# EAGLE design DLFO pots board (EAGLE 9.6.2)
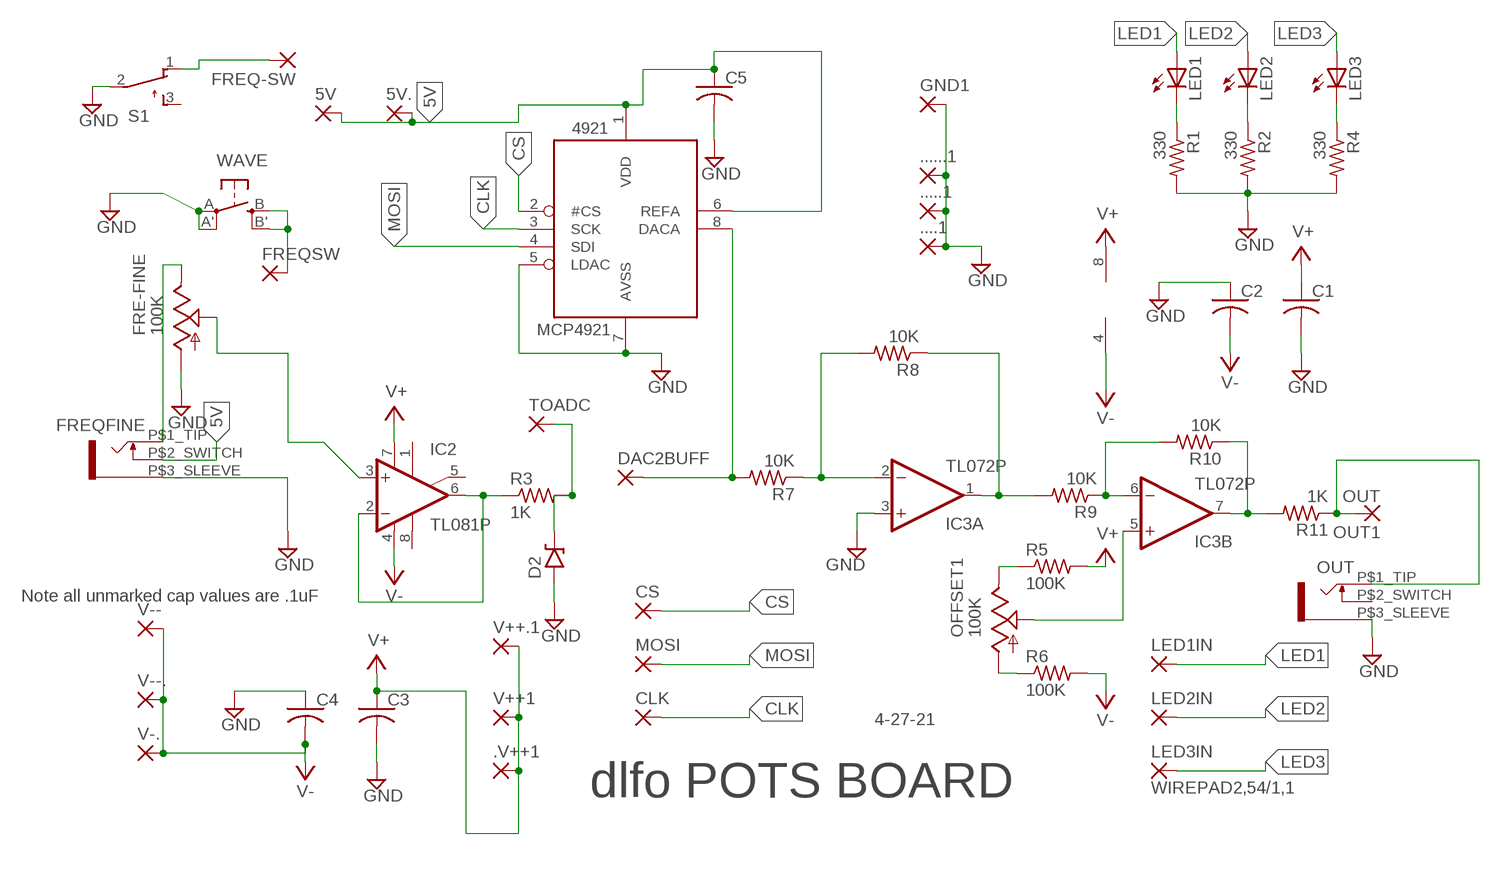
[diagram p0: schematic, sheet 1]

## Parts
5V  2,54/1,0  [2,54/1,0]
5V.  2,54/1,0  [2,54/1,0]
4921  MCP4921  [DIL08]
....1  3,17/1,3  [3,17/1,3]
.....1  3,17/1,3  [3,17/1,3]
......1  3,17/1,3  [3,17/1,3]
.V++1  2,54/1,0  [2,54/1,0]
C1  C-US025-024X044  [C025-024X044]
C2  C-US025-024X044  [C025-024X044]
C3  C-US025-024X044  [C025-024X044]
C4  C-US025-025X050  [C025-025X050]
C5  C-US025-024X044  [C025-024X044]
CLK  WIREPAD2,54/1,1  [2,54/1,1]
CS  2,54/1,0  [2,54/1,0]
D2  ZENER.2  [DO41-2]
DAC2BUFF  3,17/1,3  [3,17/1,3]
FRE-FINE  100K  9MM_SNAP-IN_POT_  [9MM_SNAP-IN_POT]
FREQ-SW  2,54/1,0  [2,54/1,0]
FREQFINE  WQP-PJ301M-12_JACK  [WQP-PJ301M-12_JACK]
FREQSW  2,54/1,0  [2,54/1,0]
GND1  3,17/1,3  [3,17/1,3]
IC2  TL081P  [DIL08@1]
IC3  TL072P  [DIL08]
LED1  LED3MM  [LED3MM]
LED1IN  2,54/1,0  [2,54/1,0]
LED2  LED3MM  [LED3MM]
LED2IN  2,54/1,0  [2,54/1,0]
LED3  LED3MM  [LED3MM]
LED3IN  WIREPAD2,54/1,1  [2,54/1,1]
MOSI  2,54/1,0  [2,54/1,0]
OFFSET1  100K  9MM_SNAP-IN_POT_  [9MM_SNAP-IN_POT]
OUT  WQP-PJ301M-12_JACK  [WQP-PJ301M-12_JACK]
OUT1  OUT  3,17/1,3  [3,17/1,3]
R1  330  R-US_0204/7  [0204/7]
R2  330  R-US_0204/7  [0204/7]
R3  1K  R-US_0204/7  [0204/7]
R4  330  R-US_0204/7  [0204/7]
R5  100K  R-US_0204/7  [0204/7]
R6  100K  R-US_0204/7  [0204/7]
R7  10K  R-US_0204/7  [0204/7]
R8  10K  R-US_0204/7  [0204/7]
R9  10K  R-US_0204/7  [0204/7]
R10  10K  R-US_0204/7  [0204/7]
R11  1K  R-US_0204/7  [0204/7]
S1  NKK-M-2012  [NKK-M-2012]
TOADC  3,17/1,3  [3,17/1,3]
V++1  2,54/1,0  [2,54/1,0]
V++.1  2,54/1,0  [2,54/1,0]
V--  2,54/1,0  [2,54/1,0]
V--.  2,54/1,0  [2,54/1,0]
V-.  2,54/1,0  [2,54/1,0]
WAVE  SPST_TACT-EVQQ2  [EVQ-Q2]

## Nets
5V: 5V.1(P) 5V..1(P) 4921.1(VDD) 4921.6(REFA) C5.1 FREQFINE.P$2_SWITCH
CLK: 4921.3(SCK) CLK.1(P)
CS: 4921.2(#CS) CS.1(P)
GND: 4921.5(LDAC) 4921.7(AVSS) ....1.1(P) .....1.1(P) ......1.1(P) C1.2 C2.1 C3.2 C4.1 C5.2 D2.A FRE-FINE.1(A) FREQFINE.P$3_SLEEVE GND1.1(P) IC3.3(A:+IN) OUT.P$3_SLEEVE R1.2 R2.2 R4.2 S1.2(P) WAVE.A'(P1) WAVE.A(P)
LED1: LED1.A LED1IN.1(P)
LED2: LED2.A LED2IN.1(P)
LED3: LED3.A LED3IN.1(P)
MOSI: 4921.4(SDI) MOSI.1(P)
N$1: D2.C R3.2 TOADC.1(P)
N$2: FREQSW.1(P) WAVE.B'(S1) WAVE.B(S)
N$3: FRE-FINE.3(E) FREQFINE.P$1_TIP
N$4: FRE-FINE.2(S) IC2.3(+IN)
N$5: IC2.2(-IN) IC2.6(OUT) R3.1
N$6: OFFSET1.3(E) R5.1
N$7: LED1.K(C) R1.1
N$8: LED2.K(C) R2.1
N$9: LED3.K(C) R4.1
N$10: IC3.1(A:OUT) R8.1 R9.2
N$11: 4921.8(DACA) DAC2BUFF.1(P) R7.2
N$12: IC3.2(A:-IN) R7.1 R8.2
N$13: IC3.5(B:+IN) OFFSET1.2(S)
N$14: IC3.6(B:-IN) R9.1 R10.2
N$15: IC3.7(B:OUT) R10.1 R11.2
N$16: OUT1.1(P) OUT.P$1_TIP R11.1
N$17: OFFSET1.1(A) R6.1
N$18: FREQ-SW.1(P) S1.1(O)
V+: .V++1.1(P) C1.1 C3.1 IC2.7(V+) IC3.8(P:V+) R5.2 V++1.1(P) V++.1.1(P)
V-: C2.2 C4.2 IC2.4(V-) IC3.4(P:V-) R6.2 V--.1(P) V--..1(P) V-..1(P)
Unconnected: IC2.1(ON1) IC2.5(ON2) IC2.8(OPT) OUT.P$2_SWITCH S1.3(S)

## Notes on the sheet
- Note all unmarked cap values are .1uF
- 4-27-21
- dlfo POTS BOARD

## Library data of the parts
5V 5V. .V++1 CS FREQ-SW FREQSW LED1IN LED2IN MOSI V++1 V++.1 V-- V--. V-. = wirepad-NONAMES:2,54/1,0: THROUGH-HOLE PAD
4921 = adafruit:MCP4921
....1 .....1 ......1 DAC2BUFF GND1 OUT1 TOADC = wirepad:3,17/1,3: THROUGH-HOLE PAD
C1-C5 = rcl:C-US: CAPACITOR, American symbol; SPICEPREFIX: C
CLK LED3IN = wirepad:WIREPAD: Wire PAD connect wire on PCB
D2 = diodes:ZENER
FRE-FINE = MusicThingModular-CL:9MM_SNAP-IN_POT: 9mm vertical snap-in pot, Alpha / Panasonic style
FREQFINE OUT = MusicThingModular-CL:WQP-PJ301M-12_JACK
IC2 = linear:TL081: OP AMP
IC3 = linear:TL072: OP AMP
LED1-LED3 = adafruit:LED: LED
OFFSET1 = MusicThingModular:9MM_SNAP-IN_POT: 9mm vertical snap-in pot, Alpha / Panasonic style
R1-R11 = rcl:R-US_: RESISTOR, American symbol
S1 = switch-CL:NKK-M-2012: NKK M2012 ON-ON SWITCH
WAVE = adafruit:SPST_TACT: SMT 6mm switch, EVQQ2 series http://www.ladyada.net/library/eagle

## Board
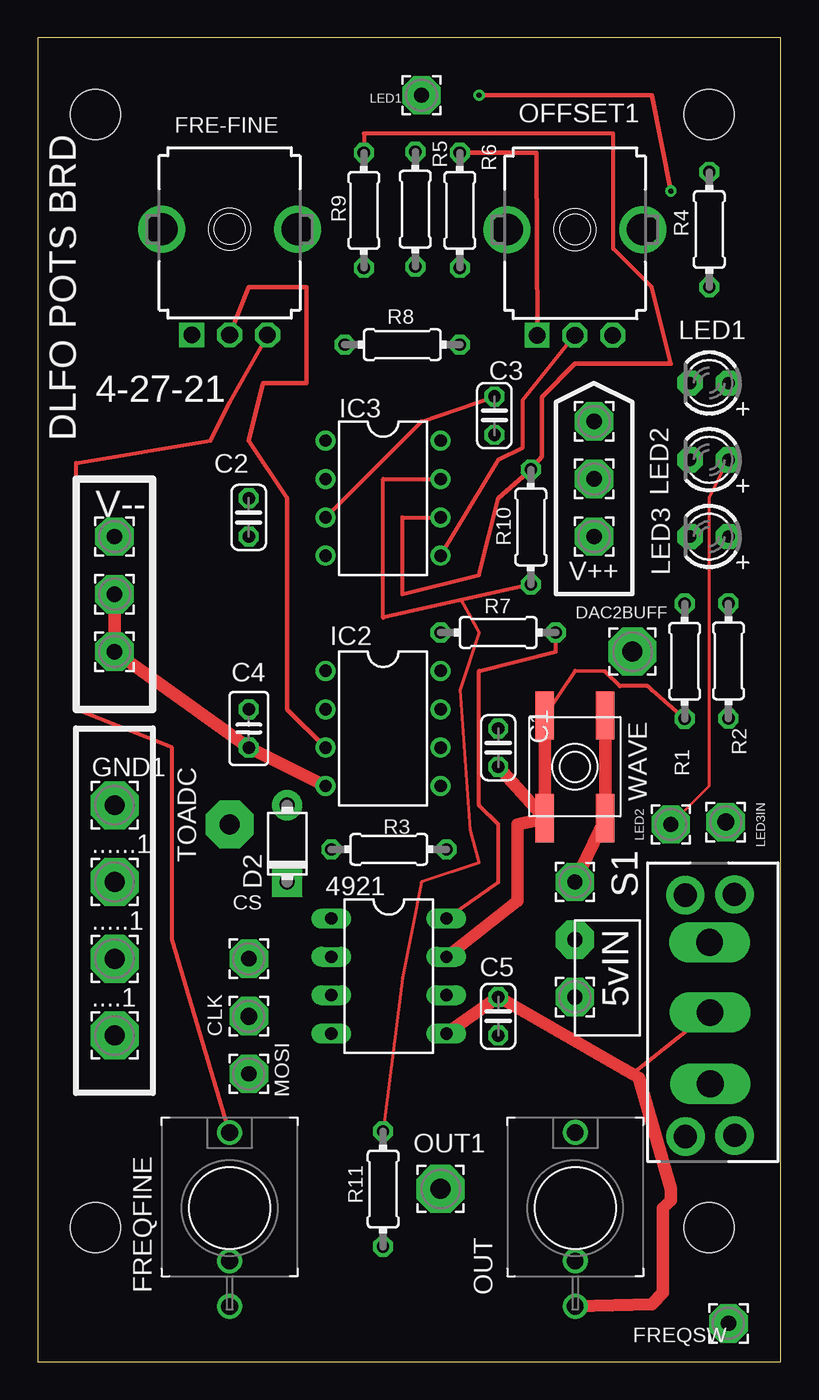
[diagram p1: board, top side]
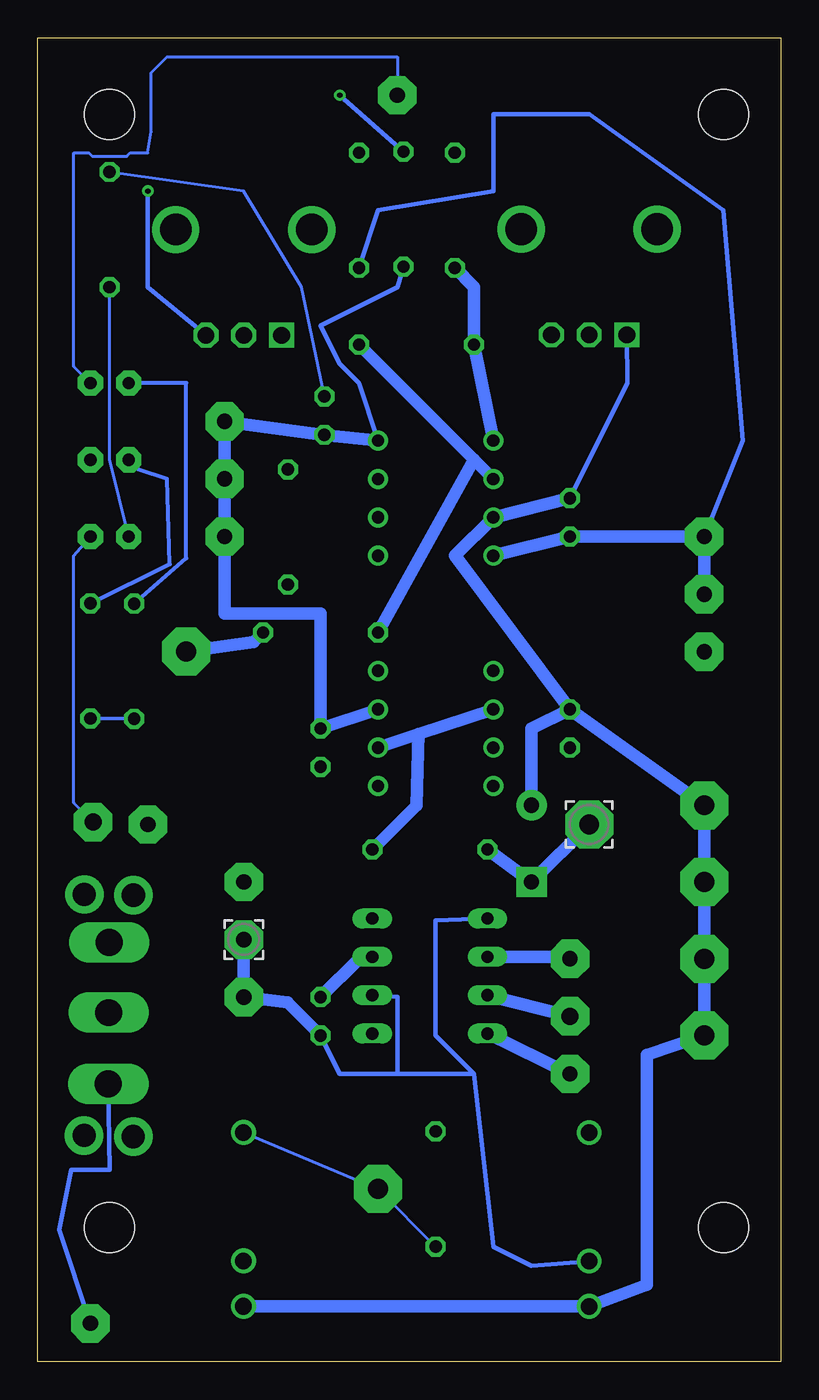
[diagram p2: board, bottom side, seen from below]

Size 49.2 x 87.62 mm. Coordinates in mm from the lower left corner, seen from the top.
Outline: 0,0 49.2,0 49.2,87.62 0,87.62 0,0
Copper layers (1*16): Top 0.035mm / dielectric 1.5mm / Bottom 0.035mm
Design rules "default": minimum track width 6mil, minimum drill 0.35mm, track to track 6mil, track to pad 6mil, pad to pad 6mil, via to via 6mil, smd to smd 6mil, copper to edge 40mil, drill to drill 6mil, minimum pad ring 10mil, minimum via ring 8mil, stop-mask expansion 4mil, vias tented up to drill 0mil, thermal gap 10mil
Holes 3.3 mm at 3.81,82.55 44.45,82.55 3.81,8.89 44.45,8.89

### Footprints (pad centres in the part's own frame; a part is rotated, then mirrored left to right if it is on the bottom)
2,54/1,0 = drill 1.016 pad 2.54 octagon: 1 0,0
DIL08 = drill 0.813 long: 1 -3.81,-3.81; 2 -1.27,-3.81; 3 1.27,-3.81; 4 3.81,-3.81; 5 3.81,3.81; 6 1.27,3.81; 7 -1.27,3.81; 8 -3.81,3.81
3,17/1,3 = drill 1.321 pad 3.175 octagon: 1 0,0
C025-024X044 = drill 0.813 octagon: 1 -1.27,0; 2 1.27,0
C025-025X050 = drill 0.813 octagon: 1 -1.27,0; 2 1.27,0
2,54/1,1 = drill 1.118 pad 2.54 octagon: 1 0,0
DO41-2 = drill 1 pad 2: A 2.54,0 | drill 1 pad 2 square: C -2.54,0
9MM_SNAP-IN_POT = drill 1.1 square: 1 -2.5,-7 | drill 1.1 octagon: 2 0,-7; 3 2.5,-7 | drill 2.1 pad 2.794: CHASSIS1 -4.5,0; CHASSIS2 4.5,0
WQP-PJ301M-12_JACK = drill 1.1: P$1_TIP 0,5; P$2_SWITCH 0,-3.5; P$3_SLEEVE 0,-6.5
DIL08@1 = drill 0.813 pad 1.27: 1 -3.81,-3.81; 2 -1.27,-3.81; 3 1.27,-3.81; 4 3.81,-3.81; 5 3.81,3.81; 6 1.27,3.81; 7 -1.27,3.81; 8 -3.81,3.81
DIL08' = drill 0.813 pad 1.27: 1 -3.81,-3.81; 2 -1.27,-3.81; 3 1.27,-3.81; 4 3.81,-3.81; 5 3.81,3.81; 6 1.27,3.81; 7 -1.27,3.81; 8 -3.81,3.81
LED3MM = drill 0.813 pad 1.676 octagon: A -1.27,0; K 1.27,0
0204/7 = drill 0.813 octagon: 1 -3.81,0; 2 3.81,0
NKK-M-2012 = drill 1.778 pad 2.286 long: 1 -5.74,-0.076; 2 -1.025,-0.051; 3 3.613,-0.025 | drill 1.524 pad 2.54: M1 -9.23,1.575; M2 6.747,1.581; M3 -9.163,-1.686; M4 6.798,-1.667
EVQ-Q2 = smd 3.2 x 1.2: A -3.4,-2; A' 3.4,-2; B -3.4,2; B' 3.4,2

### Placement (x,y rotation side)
5V  35.56,27.94 0 bottom
5V.  35.56,24.13 0 top
4921  23.24,25.53 270 top
....1  5.08,21.59 0 top
.....1  5.08,26.67 0 top
......1  5.08,31.75 0 top
.V++1  36.83,58.42 0 top
C1  30.48,40.64 270 top
C2  13.97,55.88 270 top
C3  30.23,62.61 90 top
C4  13.97,41.91 270 top
C5  30.48,22.86 90 top
CLK  13.97,22.86 0 top
CS  13.97,26.67 0 top
D2  16.51,34.29 90 top
DAC2BUFF  39.37,46.99 0 top
FRE-FINE  12.7,74.96 0 top
FREQ-SW  45.72,2.54 0 top
FREQFINE  12.7,10.16 0 top
FREQSW  35.56,31.75 0 top
GND1  5.08,36.83 0 top
IC2  22.86,41.91 270 top
IC3  TL072P  [DIL08']  22.86,57.15 270 top
LED1  44.45,64.77 180 top
LED1IN  25.4,83.82 0 top
LED2  44.45,59.69 180 top
LED2IN  41.91,35.56 0 top
LED3  44.45,54.61 180 top
LED3IN  45.54,35.71 0 top
MOSI  13.97,19.05 0 top
OFFSET1  35.56,74.93 0 top
OUT  35.59,10.17 0 top
OUT1  26.67,11.43 0 top
R1  42.82,46.35 270 top
R2  45.72,46.38 270 top
R3  23.24,33.91 180 top
R4  44.45,74.93 90 top
R5  24.99,76.28 270 top
R6  27.94,76.2 270 top
R7  30.48,48.26 0 top
R8  24.13,67.31 0 top
R9  21.59,76.2 270 top
R10  32.64,55.24 90 top
R11  22.86,11.43 90 top
S1  44.45,24.13 90 top
TOADC  12.7,35.56 90 bottom
V++1  36.83,62.23 0 top
V++.1  36.83,54.61 0 top
V--  5.08,46.99 0 top
V--.  5.08,54.61 0 top
V-.  5.08,50.8 0 top
WAVE  35.56,39.37 270 top

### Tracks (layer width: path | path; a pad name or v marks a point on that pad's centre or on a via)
5V
  Bottom 0.305: C5.1 29.21,19.05 25.4,19.05 | 25.4,19.05 20.32,19.05 | 20.32,19.05 22.86,21.59 22.86,29.21 4921.1 | 20.32,19.05 19.05,7.62 16.51,6.35 FREQFINE.P$2_SWITCH | 4921.6 25.4,24.13 25.4,19.05
  Bottom 0.813: C5.1 32.66,23.77 5V..1 5V.1
CLK
  Bottom 0.813: 4921.3 CLK.1
CS
  Bottom 0.813: 4921.2 14,26.8 CS.1
GND
  Top 0.254: IC3.3 25.4,62.23 C3.2 | R1.2 40.64,44.45 40.37,44.72 38.52,44.72 37.56,45.68 35.56,45.72 WAVE.A
  Top 0.305: S1.2 39.37,19.05
  Top 0.813: WAVE.A' C1.2 | 4921.7 31.75,30.48 31.75,35.56 WAVE.A' | WAVE.A' WAVE.A | 4921.5 C5.2 38.82,19.36 39.37,19.05 39.8,18.8 41.9,11.46 41.9,10.69 41.38,10.16 41.38,4.55 40.64,3.81 OUT.P$3_SLEEVE
  Bottom 0.203: C3.2 31.75,71.12 35.56,77.47 R4.2
  Bottom 0.254: R1.2 R2.2
  Bottom 0.305: C2.1 10.16,64.77 FRE-FINE.1
  Bottom 0.813: C4.1 GND1.1 ......1.1 .....1.1 ....1.1 8.89,20.32 8.89,5.08 FREQFINE.P$3_SLEEVE OUT.P$3_SLEEVE | C4.1 16.51,41.91 D2.A | C2.1 IC3.3 21.59,53.34 C4.1 | C5.2 27.94,26.67 4921.7
LED1
  Bottom 0.203: LED1IN.1 25.4,86.36 40.64,86.36 41.68,85.32 41.68,81.4 41.91,80.01 43.08,80.01 43.3,79.78 45.6,79.78 45.83,80.01 46.81,80.01 46.81,65.86 LED1.A
LED2
  Top 0.203: LED2IN.1 44.45,38.1 44.45,57.15 LED2.A
LED3
  Bottom 0.203: LED3IN.1 46.81,36.98 46.81,53.34 LED3.A
MOSI
  Bottom 0.813: 4921.4 MOSI.1
N$1
  Bottom 0.813: TOADC.1 D2.C R3.2
N$2
  Top 0.813: FREQSW.1 WAVE.B' WAVE.B
N$3
  Top 0.254: FREQFINE.P$1_TIP 8.89,27.94 8.89,40.64 2.54,43.18 2.54,59.48 11.43,60.96 12.7,63.5 FRE-FINE.3
N$4
  Top 0.305: IC2.3 16.51,43.18 16.51,57.15 13.97,60.96 14.92,64.77 17.78,64.77 17.78,71.12 13.97,71.12 FRE-FINE.2
N$5
  Bottom 0.813: IC2.6 24,41.53 | 24,41.53 IC2.2 | R3.1 24.13,36.83 24,41.53
N$6  (via drill 0.35)
  Top 0.305: v41.91,77.47 40.64,83.82 v29.21,83.82
  Bottom 0.305: OFFSET1.3 41.91,71.12 41.91,74.15 41.92,74.16 41.92,75.7 41.91,75.71 v41.91,77.47 | R5.1 v29.21,83.82
N$7
  Bottom 0.254: R1.1 39.37,53.18 39.37,64.77 LED1.K
N$8
  Bottom 0.254: R2.1 40.46,52.79 40.64,58.42 42.55,59.05 LED2.K
N$9
  Bottom 0.203: LED3.K 44.45,59.69 R4.1
N$10
  Bottom 0.813: IC3.1 R8.1 20.32,71.12 R9.2
N$11
  Top 0.254: 4921.8 30.48,31.75 30.48,35.56 29.21,36.83 29.21,45.72 34.29,46.99 R7.2
  Bottom 0.813: DAC2BUFF.1 34.92,47.62 R7.2
N$12
  Bottom 0.813: IC3.2 20.32,59.69 | 20.32,59.69 R8.2 | R7.1 20.32,59.69
N$13
  Top 0.254: IC3.5 30.48,59.69 32.11,60.5 32.11,63.63 OFFSET1.2
N$14
  Top 0.254: 41.91,66.04 40.64,71.12 38.1,73.66 38.1,81.28 21.59,81.28 R9.1 | 30.48,57.15 29.21,52.07 24.13,50.8 24.13,55.88 IC3.6
  Top 0.305: 41.91,66.04 35.56,66.04 33.38,63.86 33.38,59.91 R10.2 30.48,57.15
N$15
  Top 0.203: 28.03,50.4 29.21,48.26 27.94,44.45 28.63,35.2 29.21,33.02 25.4,31.75 24.13,25.4 R11.2
  Top 0.254: R10.1 28.03,50.4 22.86,49.25 22.86,58.42 IC3.7
N$16
  Bottom 0.203: OUT.P$1_TIP OUT1.1 R11.1
N$17
  Top 0.305: R6.1 33.02,80.01 OFFSET1.1
N$18
  Bottom 0.305: FREQ-SW.1 47.78,8.73 46.99,12.7 44.45,12.7 S1.1
V+
  Bottom 0.305: IC3.8 27.94,64.77 29.21,66.04 30.48,68.58 25.4,71.12 R5.2
  Bottom 0.813: IC2.7 C1.1 30.48,49.53 36.83,49.53 V++.1.1 .V++1.1 V++1.1 C3.1 IC3.8
V-
  Top 0.813: IC2.4 C4.2 V--.1 V-..1
  Bottom 0.305: V--..1 2.54,60.96 3.81,76.2 12.7,82.55 19.05,82.55 19.05,77.47 26.67,76.2 R6.2
  Bottom 0.813: IC3.4 C2.2 V--..1 V-..1

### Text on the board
tNames: LED1 | 4-27-21 | DLFO POTS BRD | V-- | V++ | LED2 | CS | 5vIN | CLK | MOSI | FREQSW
